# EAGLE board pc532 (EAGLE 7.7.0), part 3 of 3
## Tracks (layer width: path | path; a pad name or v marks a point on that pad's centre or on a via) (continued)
PDI0 (continued)
  Route2 0.305: U1.5 10.79,152.4 10.79,72.39 27.3,55.88 29.84,55.88 34.29,51.44 34.29,48.26 35.56,46.99 U16.7
  Route15 0.305: U1.5 7.62,158.12 8.89,156.84 13.97,156.84 29.21,141.6 U6.29 U7.29
PDI0P
  Top 0.305: U16.6 40.01,43.81 64.14,43.81 U20.9
PDI1
  Route2 0.305: U2.5 9.53,130.81 9.53,71.75 26.67,54.61 28.57,54.61 31.75,51.44 31.75,48.26 33.02,46.99 U16.8 | U8.29 U9.29
  Route15 0.305: U2.5 7.62,135.25 8.89,136.53 18.41,136.53 U8.29
PDI1P
  Bottom 0.305: U20.8 66.67,43.81 32.38,43.81 U16.9
PDI2
  Route2 0.305: U3.5 8.26,109.22 8.26,71.12 26.04,53.34 27.3,53.34 29.21,51.44 29.21,44.45 U16.14 | U10.29 U11.29
  Route15 0.305: U3.5 7.62,112.39 8.89,113.67 26.04,113.67 U10.29
PDI2P
  Route2 0.305: U16.15 40.01,36.2 81.92,36.2 U20.23
PDI3
  Route2 0.305: U16.13 25.4,45.72 25.4,52.07 6.99,70.48 6.99,87.63 U4.5 | U12.29 U13.29
  Route15 0.305: U12.29 24.77,90.81 8.89,90.81 7.62,89.53 U4.5
PDI3P
  Bottom 0.305: U20.7 65.41,40.01 32.38,40.01 U16.12
PDO0
  Route2 0.305: U1.4 3.81,159.38 3.81,121.28 RES1.2 | U7.26 U6.26
  Route15 0.305: U1.4 7.62,160.66 8.89,159.38 13.97,159.38 29.84,143.51 34.29,143.51 U6.26
PDO1
  Route2 0.305: U8.26 U9.26
  Route15 0.305: U8.26 34.29,128.27 29.21,128.27 19.68,137.79 15.24,137.79 13.97,139.06 6.35,139.06 U2.4 3.81,136.53 3.81,118.75 RES1.3
PDO2
  Route2 0.305: RES1.4 U3.4 | U10.26 U11.26
  Route15 0.305: U3.4 7.62,114.94 8.89,116.2 14.61,116.2 15.88,114.94 32.38,114.94 U10.26
PDO3
  Top 0.305: U12.26 34.29,97.79 15.88,97.79 13.97,95.89 10.79,95.89 6.99,92.08 U4.4
  Route2 0.305: RES1.6 2.54,94.61 U4.4 | U12.26 U13.26
Q0
  Bottom 0.305: U22.1 95.25,160.02 U22.13 93.98,156.21 108.58,156.21 117.47,147.32 121.92,147.32 125.73,143.51 125.73,139.7 U27.4
Q1
  Top 0.305: U22.11 90.17,160.02 U22.3
  Bottom 0.305: U27.7 118.11,139.7 118.11,142.88 107.31,153.67 91.44,153.67 U22.11
Q2
  Top 0.305: U22.9 85.09,160.02 U22.5
  Bottom 0.305: U22.9 86.36,153.67 86.36,151.76 87,151.13 107.31,151.13 115.57,142.88 115.57,137.16 120.65,132.08 U27.9
Q3
  Top 0.305: U21.9 83.82,171.45 86.36,171.45 U21.11
  Bottom 0.305: U27.12 124.46,130.81 124.46,137.16 120.65,140.97 120.65,142.88 108.58,154.94 92.71,154.94 91.44,156.21 91.44,166.37 U21.11
Q4
  Top 0.305: U17.13 72.39,160.02 U17.1
  Bottom 0.305: U28.4 127,125.73 119.38,125.73 118.11,127 118.11,132.72 114.3,136.53 114.3,142.88 107.31,149.86 80.01,149.86 74.93,154.94 72.39,154.94 U17.13
Q5
  Top 0.305: U17.11 67.31,160.02 U17.3
  Bottom 0.305: U17.11 68.58,153.67 68.58,151.13 71.12,148.59 107.31,148.59 113.03,142.88 113.03,134.62 116.84,130.81 116.84,125.73 118.11,124.46 120.65,124.46 U28.7
Q6
  Top 0.305: U17.9 62.23,160.02 U17.5
  Bottom 0.305: U28.9 120.65,117.47 114.3,123.83 114.3,125.73 104.14,135.89 104.14,141.6 100.97,144.78 67.31,144.78 66.04,146.05 66.04,148.59 63.5,151.13 63.5,153.67 U17.9
Q7
  Top 0.305: U5.13 49.53,160.02 U5.1
  Bottom 0.305: U28.12 123.19,119.38 120.65,119.38 115.57,124.46 115.57,130.18 111.76,133.99 111.76,142.88 108.58,146.05 69.22,146.05 68.58,146.69 68.58,148.59 66.04,151.13 66.04,153.67 63.5,156.21 63.5,158.75 62.23,160.02 49.53,160.02 U5.13
Q8
  Top 0.305: U5.11 44.45,160.02 U5.3
  Bottom 0.305: U5.11 44.45,154.94 59.69,154.94 60.96,153.67 60.96,151.76 63.5,149.22 63.5,146.05 66.04,143.51 100.33,143.51 102.87,140.97 102.87,135.89 113.03,125.73 113.03,119.38 120.65,111.76 128.27,111.76 U29.4
Q9
  Top 0.305: U5.9 39.37,160.02 U5.5
  Bottom 0.305: U29.7 121.92,110.49 119.38,110.49 111.76,118.11 111.76,120.65 104.78,127.64 104.78,132.08 99.06,137.79 65.41,137.79 63.5,139.7 63.5,142.88 60.96,145.41 60.96,148.59 59.69,149.86 44.45,149.86 U5.9
Q10
  Top 0.305: U18.13 69.85,62.23 67.31,62.23 U18.11
  Bottom 0.305: U18.11 59.69,69.85 59.69,72.39 62.23,74.93 88.9,74.93 97.79,83.82 100.97,83.82 118.75,101.6 U29.9
QA0
  Top 0.305: RES8.1 97.79,160.02 U22.2
QA1
  Route2 0.305: RES8.3 92.71,153.67 91.44,154.94 90.17,154.94 88.9,156.21 88.9,163.83 U22.4
QA2
  Route2 0.305: RES8.5 87.63,153.67 86.36,154.94 85.09,154.94 83.82,156.21 83.82,163.83 U22.6
QA3
  Route2 0.305: U21.10 81.28,166.37 81.28,161.29 78.74,158.75 78.74,156.21 80.01,154.94 81.28,154.94 82.55,153.67 RES8.7
QA4
  Route2 0.305: RES5.1 74.93,153.67 73.66,154.94 73.66,161.29 U17.2
QA5
  Route2 0.305: RES5.3 66.04,156.21 66.04,163.83 U17.4
QA6
  Route2 0.305: RES5.5 60.96,156.21 60.96,163.83 U17.6
QA7
  Route2 0.305: RES5.7 55.88,156.21 55.88,157.48 50.8,162.56 49.53,162.56 U5.2
QA8
  Route2 0.305: RES2.1 43.18,156.21 43.18,163.83 U5.4
QA9
  Route2 0.305: RES2.5 38.1,151.13 38.1,163.83 U5.6
QA10
  Top 0.305: U18.12 67.31,64.77 67.31,78.74 RES7.1
QB0
  Route2 0.305: RES9.1 97.79,149.86 96.52,151.13 96.52,153.67 93.98,156.21 91.44,156.21 U22.12
QB1
  Route2 0.305: RES9.3 92.71,149.86 91.44,151.13 91.44,153.67 90.17,153.67 87.63,156.21 86.36,156.21 U22.10
QB2
  Route2 0.305: RES9.5 87.63,149.86 86.36,151.13 86.36,153.03 85.72,153.67 85.09,153.67 82.55,156.21 81.28,156.21 U22.8
QB3
  Route2 0.305: RES9.7 82.55,149.86 81.28,151.13 81.28,153.67 80.01,153.67 77.47,156.21 77.47,158.75 78.74,160.02 78.74,166.37 80.01,167.64 U21.8
QB4
  Route2 0.305: RES6.1 74.93,149.86 73.66,151.13 73.66,153.67 71.12,156.21 68.58,156.21 U17.12
QB5
  Route2 0.305: RES6.3 66.04,151.13 66.04,154.94 64.77,156.21 63.5,156.21 U17.10
QB6
  Route2 0.305: RES6.5 60.96,151.13 60.96,153.67 U17.8
QB7
  Route2 0.305: RES6.7 53.34,153.67 48.26,153.67 U5.12
QB8
  Route2 0.305: RES2.3 39.37,154.94 U5.10
QB9
  Route2 0.305: RES2.7 34.29,149.86 U5.8
QB10
  Top 0.305: RES7.3 62.23,78.74 62.23,64.77 U18.10
QF0
  Top 0.305: U32.2 132.08,72.39 124.46,72.39 U32.6
QF1
  Route2 0.305: U32.8 121.92,62.23 129.54,62.23 U32.12
QO0
  Bottom 0.305: U19.9 68.58,55.88 104.78,55.88 117.47,68.58 123.19,68.58 U32.5
QO1
  Bottom 0.305: U19.10 67.31,54.61 105.41,54.61 112.39,61.59 121.28,61.59 U32.9
QRA0
  Route2 0.305: U12.4 93.98,96.52 93.98,109.22 U10.4 93.98,111.76 93.98,124.46 U8.4 93.98,127 93.98,139.7 U6.4 96.52,144.78 96.52,149.86 95.25,151.13 RES8.2
QRA1
  Route2 0.305: U12.5 90.17,96.52 91.44,97.79 91.44,107.95 90.17,109.22 U10.5 90.17,111.76 91.44,113.03 91.44,123.19 90.17,124.46 U8.5 90.17,127 91.44,128.27 91.44,138.43 90.17,139.7 U6.5 90.17,144.78 91.44,146.05 91.44,149.86 90.17,151.13 RES8.4
QRA2
  Route2 0.305: U12.7 86.36,96.52 86.36,109.22 U10.7 86.36,111.76 86.36,124.46 U8.7 86.36,127 86.36,138.43 85.09,139.7 U6.7 85.09,144.78 86.36,146.05 86.36,149.86 85.09,151.13 RES8.6
QRA3
  Route2 0.305: U12.8 82.55,96.52 83.82,97.79 83.82,107.95 82.55,109.22 U10.8 82.55,111.76 83.82,113.03 83.82,123.19 82.55,124.46 U8.8 82.55,127 83.82,128.27 83.82,138.43 82.55,139.7 U6.8 82.55,144.78 81.28,146.05 81.28,149.86 80.01,151.13 RES8.8
QRA4
  Route2 0.305: U12.11 76.2,96.52 76.2,109.22 U10.11 76.2,111.76 76.2,124.46 U8.11 76.2,127 76.2,138.43 74.93,139.7 U6.11 74.93,144.78 73.66,146.05 73.66,149.86 72.39,151.13 RES5.2
QRA5
  Route2 0.305: U12.12 72.39,96.52 73.66,97.79 73.66,107.95 72.39,109.22 U10.12 72.39,111.76 73.66,113.03 73.66,123.19 72.39,124.46 U8.12 72.39,127 73.66,128.27 73.66,138.43 72.39,139.7 U6.12 72.39,143.51 71.12,144.78 71.12,148.59 RES5.4
QRA6
  Route2 0.305: U12.14 68.58,96.52 68.58,109.22 U10.14 68.58,111.76 68.58,124.46 U8.14 68.58,127 68.58,138.43 67.31,139.7 U6.14 67.31,143.51 66.04,144.78 66.04,148.59 RES5.6
QRA7
  Route2 0.305: U12.15 64.77,96.52 66.04,97.79 66.04,106.68 64.77,107.95 U10.15 64.77,111.76 66.04,113.03 66.04,121.92 64.77,123.19 U8.15 64.77,127 66.04,128.27 66.04,138.43 64.77,139.7 U6.15 64.77,142.24 60.96,146.05 60.96,148.59 RES5.8
QRA8
  Route2 0.305: U12.17 60.96,96.52 60.96,109.22 U10.17 60.96,111.76 60.96,124.46 U8.17 60.96,127 60.96,138.43 59.69,139.7 U6.17 59.69,142.24 55.88,146.05 50.8,146.05 RES2.2
QRA9
  Route2 0.305: U12.18 57.15,96.52 58.42,97.79 58.42,107.95 57.15,109.22 U10.18 57.15,111.76 58.42,113.03 58.42,123.19 57.15,124.46 U8.18 57.15,127 58.42,128.27 58.42,138.43 57.15,139.7 U6.18 54.61,143.51 43.18,143.51 RES2.6
QRA10
  Route2 0.305: U8.19 54.61,124.46 55.88,123.19 55.88,113.03 54.61,111.76 U10.19 54.61,108.58 55.88,107.31 55.88,98.42 54.61,97.16 U12.19 54.61,90.81 55.88,89.53 55.88,87 60.33,82.55 63.5,82.55 RES7.2
  Route15 0.305: U8.19 55.88,127 55.88,139.7 U6.19
QRB0
  Route2 0.305: U13.4 92.71,92.71 91.44,93.98 91.44,95.89 92.71,97.16 U11.4 92.71,107.95 91.44,109.22 91.44,111.76 92.71,113.03 U9.4 92.71,123.19 91.44,124.46 91.44,127 92.71,128.27 U7.4 92.71,138.43 91.44,139.7 91.44,143.51 RES9.2
QRB1
  Route2 0.305: U13.5 90.17,92.71 88.9,93.98 88.9,96.52 90.17,97.79 U11.5 90.17,107.95 88.9,109.22 88.9,111.76 90.17,113.03 U9.5 90.17,123.19 88.9,124.46 88.9,127 90.17,128.27 U7.5 88.9,134.62 88.9,146.05 RES9.4
QRB2
  Route2 0.305: U13.7 85.09,92.71 83.82,93.98 83.82,96.52 85.09,97.79 U11.7 85.09,107.95 83.82,109.22 83.82,111.76 85.09,113.03 U9.7 85.09,123.83 83.82,125.09 83.82,127 85.09,128.27 U7.7 85.09,138.43 83.82,139.7 83.82,146.05 RES9.6
QRB3
  Route2 0.305: U13.8 82.55,92.71 81.28,93.98 81.28,97.79 82.55,99.06 U11.8 82.55,107.95 81.28,109.22 81.28,111.76 82.55,113.03 U9.8 82.55,123.19 81.28,124.46 81.28,127 82.55,128.27 U7.8 81.28,134.62 81.28,143.51 80.01,144.78 RES9.8
QRB4
  Route2 0.305: U13.11 74.93,92.71 73.66,93.98 73.66,96.52 74.93,97.79 U11.11 74.93,107.95 73.66,109.22 73.66,111.76 74.93,113.03 U9.11 74.93,123.19 73.66,124.46 73.66,127 74.93,128.27 U7.11 74.93,138.43 73.66,139.7 73.66,143.51 72.39,144.78 RES6.2
QRB5
  Route2 0.305: U13.12 72.39,92.71 71.12,93.98 71.12,96.52 72.39,97.79 U11.12 72.39,107.95 71.12,109.22 71.12,111.76 72.39,113.03 U9.12 72.39,123.19 71.12,124.46 71.12,127 72.39,128.27 U7.12 71.12,134.62 71.12,143.51 RES6.4
QRB6
  Route2 0.305: U13.14 67.31,92.71 66.04,93.98 66.04,96.52 67.31,97.79 U11.14 67.31,107.95 66.04,109.22 66.04,111.76 67.31,113.03 U9.14 67.31,123.19 66.04,124.46 66.04,127 67.31,128.27 U7.14 67.31,138.43 66.04,139.7 66.04,142.24 62.23,146.05 RES6.6
QRB7
  Route2 0.305: U13.15 64.77,92.71 63.5,93.98 63.5,96.52 64.77,97.79 U11.15 63.5,104.14 63.5,111.76 64.77,113.03 U9.15 63.5,119.38 63.5,127 64.77,128.27 U7.15 63.5,134.62 63.5,142.24 59.69,146.05 58.42,146.05 RES6.8
QRB8
  Route2 0.305: U13.17 59.69,92.71 58.42,93.98 58.42,96.52 59.69,97.79 U11.17 59.69,107.95 58.42,109.22 58.42,111.76 59.69,113.03 U9.17 59.69,123.19 58.42,124.46 58.42,127 59.69,128.27 U7.17 59.69,138.43 58.42,139.7 58.42,142.24 55.88,144.78 46.99,144.78 RES2.4
QRB9
  Route2 0.305: U13.18 57.15,92.71 55.88,93.98 55.88,96.52 57.15,97.79 U11.18 57.15,107.95 55.88,109.22 55.88,111.76 57.15,113.03 U9.18 57.15,123.19 55.88,124.46 55.88,127 57.15,128.27 U7.18 53.34,137.16 53.34,141.6 52.7,142.24 39.37,142.24 RES2.8
QRB10
  Route2 0.305: RES7.4 54.61,86.36 U13.19 53.34,88.9 53.34,100.33 54.61,101.6 U11.19 53.34,104.14 53.34,115.57 54.61,116.84 U9.19 53.34,119.38 53.34,128.27 54.61,129.54 U7.19
RFRQ
  Route2 0.305: U50.11 234.95,87.63 230.5,87.63 227.33,84.45 227.33,77.47 221.62,71.75 221.62,69.85 220.98,69.22 U46.29
RFRQS
  Route15 0.305: U50.12 237.49,87.63 186.06,87.63 183.51,90.17 170.18,90.17 U39.5
RST_JFILT
  Bottom 0.305: C47.+ D2.A R1.1 R2.2 U42.1
RST_JIN
  Route15 0.305: J3.1 234.95,115.57 234.95,153.67 231.14,157.48 231.14,176.53 219.71,187.96 219.71,190.5 214.63,195.58 214.63,203.2 R2.1
RSTO
  Route2 0.305: CONN12.B2 314.96,210.82 313.69,209.55 | 313.69,209.55 313.69,196.85 314.96,195.58 CONN13.B2 314.96,190.5 313.69,189.23 313.69,176.53 314.96,175.26 CONN14.B2 314.96,170.18 313.69,168.91 313.69,156.21 314.96,154.94 CONN15.B2 313.69,151.13 313.69,57.78 309.25,53.34 299.08,53.34 297.18,51.44 297.18,49.53 299.72,46.99 299.72,44.45 U60.38 | 313.69,209.55 312.42,210.82 236.22,210.82 227.33,201.93 226.06,201.93 U42.2
  Route15 0.305: U48.38 199.39,41.91 231.14,41.91 U52.38 233.68,41.91 265.43,41.91 U55.38 267.97,41.91 299.72,41.91 U60.38
  Bottom 0.305: U42.2 U42.3
RTS0
  Top 0.305: U47.7 195.58,60.96 217.17,60.96 218.44,59.69 218.44,57.15 CONN3.4
RTS1
  Top 0.305: U49.7 195.58,25.4 212.09,25.4 214,27.3 217.81,27.3 218.44,26.67 218.44,24.13 CONN4.4
RTS2
  Top 0.305: U51.7 229.87,60.96 251.46,60.96 252.73,59.69 252.73,57.15 CONN5.4
RTS3
  Top 0.305: U53.7 229.87,25.4 246.38,25.4 248.28,27.3 252.09,27.3 252.73,26.67 252.73,24.13 CONN6.4
RTS4
  Bottom 0.305: CONN7.4 287.02,54.61 265.43,54.61 U54.7
RTS5
  Top 0.305: U56.7 264.16,25.4 280.67,25.4 282.57,27.3 286.38,27.3 287.02,26.67 287.02,24.13 CONN8.4
RTS6
  Top 0.305: U59.7 298.45,60.96 320.04,60.96 321.31,59.69 321.31,57.15 CONN9.4
RTS7
  Top 0.305: U61.7 298.45,25.4 314.96,25.4 316.87,27.3 320.68,27.3 321.31,26.67 321.31,24.13 CONN10.4
RXD0
  Top 0.305: U47.2 207.01,57.15 215.9,57.15 CONN3.3
RXD1
  Top 0.305: U49.2 207.01,21.59 215.9,21.59 CONN4.3
RXD2
  Top 0.305: U51.2 241.3,57.15 250.19,57.15 CONN5.3
RXD3
  Top 0.305: U53.2 241.3,21.59 250.19,21.59 CONN6.3
RXD4
  Top 0.305: U54.2 275.59,57.15 284.48,57.15 CONN7.3
RXD5
  Top 0.305: U56.2 275.59,21.59 284.48,21.59 CONN8.3
RXD6
  Top 0.305: U59.2 309.88,57.15 318.77,57.15 CONN9.3
RXD7
  Top 0.305: U61.2 309.88,21.59 318.77,21.59 CONN10.3
SCSI0
  Route15 0.305: U40.13 U41.22
SCSICLK
  Route2 0.305: U34.8 124.46,41.91 140.34,41.91 142.88,44.45 167.64,44.45 U41.20
SCSII
  Route2 0.305: U38.8 156.21,105.41 154.94,104.14 154.94,69.85 157.48,67.31 175.26,67.31 177.8,64.77 177.8,53.34 176.53,52.07 U40.19
SCSII1  (via drill 0.33)
  Top 0.305: v224.79,72.39 v224.79,62.23 | U46.9 229.87,85.09 269.24,85.09 U57.26
  Route2 0.305: v224.79,72.39 228.6,76.2 U46.9
  Route15 0.305: U40.2 177.8,59.69 184.15,59.69 185.42,60.96 223.52,60.96 v224.79,62.23
SELECT
  Route2 0.305: U40.5 166.37,60.96 158.75,60.96 RES13.12
  Route15 0.305: RES13.12 160.02,67.31 221.62,67.31 222.25,67.94 222.25,72.39 227.33,77.47 234.95,77.47 U46.4
ST0
  Bottom 0.305: U35.S8 190.5,166.37 190.5,164.47 189.87,163.83 175.26,163.83 172.72,166.37 149.86,166.37 147.32,168.91 132.08,168.91 130.81,170.18 130.81,172.72 U24.K8
ST1  (via drill 0.33)
  Route15 0.305: U35.S7 191.77,165.1 205.74,151.13 228.6,151.13 230.5,149.22 v230.5,145.41
  Bottom 0.305: U46.3 245.11,82.55 250.19,82.55 250.82,83.19 250.82,97.16 234.95,113.03 234.95,133.99 230.5,138.43 v230.5,145.41 | U35.S7 187.96,166.37 179.07,166.37 175.26,170.18 169.54,170.18 168.28,171.45 149.86,171.45 148.59,172.72 133.35,172.72 U24.K9
ST2
  Bottom 0.305: U24.L8 129.54,170.18 132.08,167.64 146.05,167.64 149.86,163.83 172.72,163.83 175.26,161.29 187.96,161.29 U35.S6
ST4
  Bottom 0.305: U24.L9 133.35,170.18 148.59,170.18 149.86,168.91 172.72,168.91 176.53,165.1 U35.N7
STERM
  Bottom 0.813: D3.C CONN16.26
STERM0
  Bottom 0.813: D1.C CONN1.26
STS0
  Top 0.305: RES15.7 167.64,15.24 167.64,12.7 168.91,11.43 LED1.1
STS1
  Bottom 0.305: LED2.1 171.45,11.43 RES16.7
STS2
  Bottom 0.305: LED3.1 172.72,11.43 172.72,15.24 RES15.5
STS3
  Bottom 0.305: LED4.1 176.53,10.79 173.99,13.34 RES16.5
STS4
  Bottom 0.305: CONN2.7 182.25,10.16 180.34,12.06 180.34,15.24 RES15.3
STS5
  Top 0.305: CONN2.5 184.78,12.06 180.97,12.06 RES16.3
STS6
  Bottom 0.305: CONN2.3 189.23,11.43 RES15.1
STS7
  Top 0.305: CONN2.1 187.96,13.97 RES16.1
SWAP
  Route2 0.305: U37.6 163.83,123.19 175.26,123.19 176.53,121.92 176.53,86.36 RES13.3
  Bottom 0.305: U46.11 222.25,85.09 185.42,85.09 182.88,82.55 171.45,82.55 161.29,72.39 RES13.3
TXD0
  Top 0.305: U47.3 205.74,55.88 214.63,55.88 CONN3.5
TXD1
  Top 0.305: U49.3 205.74,20.32 CONN4.5
TXD2
  Top 0.305: U51.3 240.03,55.88 248.92,55.88 CONN5.5
TXD3
  Top 0.305: U53.3 240.03,20.32 CONN6.5
TXD4
  Top 0.305: U54.3 274.32,55.88 283.21,55.88 CONN7.5
TXD5
  Top 0.305: U56.3 274.32,20.32 CONN8.5
TXD6
  Top 0.305: U59.3 308.61,55.88 317.5,55.88 CONN9.5
TXD7
  Top 0.305: U61.3 308.61,20.32 CONN10.5

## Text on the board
Top: 1 | PC532 Motherboard / (C) 1989 Rev 1D+ / G.Scolaro/D.Rand
Route2: 2
Ground: 3
Power: 4
Route15: 5
Bottom: 6
tPlace: 1 | 2 | 25 | 1 | 3 | 50 | 2 | 1 | 2 | 3 | 1 | 1 | 1 | 1 | 1 | 1 | 1 | 1 | 25 | 1 | 1 | 50 | 2 | Disk & Tape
